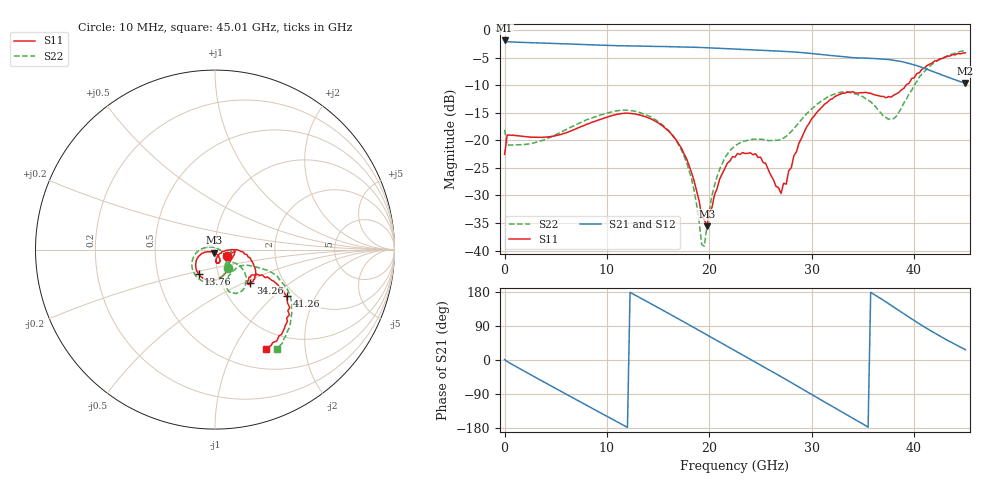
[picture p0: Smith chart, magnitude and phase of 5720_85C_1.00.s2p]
! Device:  ADRF5720
! Description: 0.5dB LSB GaAs MMIC 6-bit Digital Attenuator
! Frequency:  0.000009 -  40 GHz
! Ports:
!	RF1	= Port 1
!	RF2	= Port 2
! Vdd:  3.3 Volt
! Vss:  -3.3 Volt
! Control:  0/3.3 Volt
! State:  1.00 dB attenuation
! Data:  The device was measured using G-S-G Probes on a matrix board.
!  Data was collected using an calibrated 4 port network analyzer.
!  The reference plane for this measurement is at the launchers.
! Note:  Analog Devices supplies this data as a sample of measured data
!  for this product.  Your particular data for this product may vary.
!  Data was taken at 85 degrees C.
!  Analog Devices reserves the right to change this data at anytime.
# GHZ S DB R 45.0
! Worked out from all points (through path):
!   181 points, 10 MHz to 45.01 GHz, reference 45 ohm
!   highest |S21| = -1.86 dB at 10 MHz (marker M1); lowest = -9.6 dB at 45.01 GHz (marker M2)
!   group delay of S21, straight-line fit = 42.7 ps
!   lowest |S11| = -35.6 dB at 19.76 GHz (marker M3), VSWR 1.03, Z = 44.7 - j1.45 ohm
!   |S11| at or under -10 dB: start of sweep to 39.21 GHz
!   |S22| runs from -39.2 to -3.7 dB; largest |S21 - S12| = 0.0042
!   S11 on the Smith chart (normalised r, x): 10 MHz: 1.14, -0.08; 13.76 GHz: 0.80, -0.23; 34.26 GHz: 1.37, -0.54; 41.26 GHz: 1.81, -1.22; 45.01 GHz: 0.75, -1.36
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0.01  -22.54 -26.4  -1.86 1.2  -1.85 1.3  -18.07 -54.9
0.26  -19.04 -4.7  -2.09 -4.0  -2.08 -4.0  -20.88 -5.0
4.01  -19.39 -38.1  -2.35 -60.5  -2.33 -60.4  -19.79 -41.5
5.76  -18.76 -48.4  -2.46 -86.4  -2.45 -86.3  -18.28 -55.8
7.76  -17.31 -61.1  -2.60 -115.8  -2.58 -115.7  -16.47 -72.2
10.76  -15.36 -89.6  -2.80 -159.6  -2.78 -159.5  -14.70 -101.7
13.76  -15.68 -123.8  -2.91 156.5  -2.89 156.7  -15.31 -135.0
15.26  -17.17 -141.0  -2.95 134.3  -2.93 134.4  -16.94 -153.1
17.76  -23.24 -163.6  -3.05 96.8  -3.03 97.0  -23.89 172.4
18.51  -27.32 -164.4  -3.08 85.5  -3.06 85.7  -29.03 155.4
19.26  -33.79 -143.2  -3.14 74.1  -3.12 74.3  -38.91 101.7
19.51  -34.40 -126.9  -3.15 70.3  -3.14 70.5  -39.21 53.6
19.76  -35.60 -102.1  -3.18 66.5  -3.16 66.7  -35.75 17.6
21.01  -27.04 -61.1  -3.28 47.5  -3.26 47.8  -25.25 -26.1
22.76  -22.37 -70.2  -3.45 21.0  -3.42 21.3  -20.70 -46.8
25.01  -23.05 -84.0  -3.65 -13.1  -3.62 -12.9  -19.80 -60.2
27.01  -29.65 -42.7  -3.82 -44.0  -3.80 -43.7  -19.82 -45.0
30.26  -15.54 -8.6  -4.29 -95.2  -4.26 -94.9  -13.90 -36.8
34.26  -11.39 -42.9  -5.02 -157.3  -5.00 -157.0  -11.58 -66.4
37.76  -12.14 -34.9  -5.39 144.4  -5.37 144.7  -16.07 -45.7
41.26  -6.42 -33.0  -7.10 83.0  -7.07 83.4  -7.03 -27.7
45.01  -4.11 -62.6  -9.63 27.2  -9.59 27.6  -3.67 -58.1
